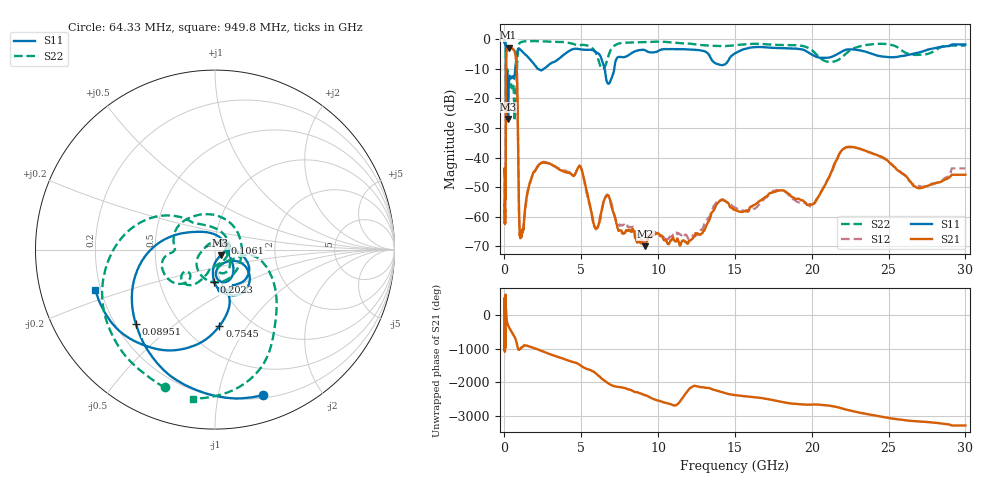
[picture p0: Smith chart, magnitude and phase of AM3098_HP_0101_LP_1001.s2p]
! Date/Time: Thu, Feb 28, 2019 8:36 AM
! Network Analyzer: Agilent Technologies E8364B Rev: A.07.50.67
! Sweep from 0.010 to 30.000 GHz, 1601 Points, Sweep Type: LOG
! Power Supply: 5.022 V, 0.001 A
# Hz S DB R 50
!freq MagS11 AngS11 MagS21 AngS21 MagS12 AngS12 MagS22 AngS22
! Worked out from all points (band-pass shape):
!   1601 points, 10 MHz to 30 GHz, reference 50 ohm
!   highest |S21| = -2.79 dB at 267.8 MHz (marker M1); lowest = -70.0 dB at 9.164 GHz (marker M2)
!   |S21| within 3 dB of the highest: 114.4 MHz to 735.6 MHz (621.2 MHz wide, 146 % of centre)
!   lowest |S11| = -26.9 dB at 236.3 MHz (marker M3), VSWR 1.09, Z = 53.1 - j3.44 ohm
!   |S11| at or under -10 dB: 97.45 MHz to 701.8 MHz (604.4 MHz wide, 151 % of centre); 2.19 GHz to 2.546 GHz (355.9 MHz wide, 15 % of centre); 6.522 GHz to 7.145 GHz (622.4 MHz wide, 9.11 % of centre)
!   |S22| runs from -27.6 to -0.5 dB; largest |S21 - S12| = 0.01
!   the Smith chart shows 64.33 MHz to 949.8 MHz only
!   S11 on the Smith chart (normalised r, x): 64.33 MHz: 0.23, -1.36; 89.51 MHz: 0.28, -0.37; 106.1 MHz: 1.12, +0.08; 202.3 MHz: 0.93, -0.35; 754.5 MHz: 0.72, -0.75; 949.8 MHz: 0.18, -0.16
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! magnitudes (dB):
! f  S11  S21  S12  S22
! 10 MHz  -0.3  -44.9  -46.6  -0.6
! 38.04 MHz  -0.5  -62.1  -61.0  -0.9
! 64.33 MHz  -1.4  -53.1  -53.0  -1.8
! 80.58 MHz  -2.4  -53.0  -50.9  -2.9
! 89.51 MHz  -4.4  -34.4  -34.4  -4.8
! 106.1 MHz  -23.6  -8.2  -8.2  -20.7
! 144.7 MHz  -17.7  -3.7  -3.6  -13.8
! 202.3 MHz  -14.8  -3.1  -3.1  -10.9
! 236.3 MHz  -26.9  -2.9  -2.9  -12.5
! 267.8 MHz  -17.9  -2.8  -2.8  -13.0
! 550.5 MHz  -12.5  -3.3  -3.3  -14.8
! 754.5 MHz  -7.4  -6.6  -6.6  -21.3
! 838.1 MHz  -4.1  -17.0  -17.0  -7.2
! 949.8 MHz  -3.0  -58.5  -59.1  -1.5
! 2.084 GHz  -9.4  -43.6  -43.7  -0.6
! 4.903 GHz  -3.3  -42.9  -42.7  -1.9
! 5.929 GHz  -4.2  -64.1  -64.2  -4.3
! 7.926 GHz  -5.8  -64.6  -62.9  -1.1
! 9.164 GHz  -3.7  -70.0  -68.8  -0.9
! 19.8 GHz  -4.5  -56.0  -56.3  -2.9
! 22.67 GHz  -3.4  -36.4  -36.6  -3.2
! 30 GHz  -1.7  -45.9  -43.7  -2.0
